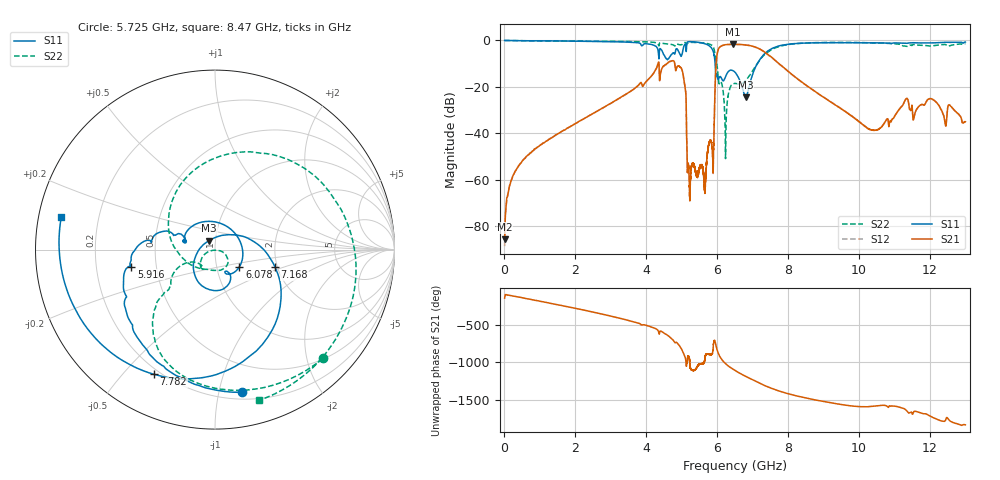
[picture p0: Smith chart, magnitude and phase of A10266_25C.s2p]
!Akoustis s2p Touchstone File
!Script Version: 1.0
!Creation Data: 12/28/2021 at 11:15 AM
!DEEMBEDDING STATE: ON
!DEMBEDDING OFFSET: 0.4 dB static
! Freq Mag(S11) Angle(S11)Mag(S21) Angle(S21)Mag(S12) Angle(S12)Mag(S22) Angle(S22)
# GHz S MA R 50
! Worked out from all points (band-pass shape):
!   11000 points, 10 MHz to 13 GHz, reference 50 ohm
!   highest |S21| = -1.69 dB at 6.448 GHz (marker M1); lowest = -85.7 dB at 10 MHz (marker M2)
!   |S21| within 3 dB of the highest: 6.019 GHz to 7.311 GHz (1.292 GHz wide, 19.4 % of centre)
!   lowest |S11| = -24.5 dB at 6.805 GHz (marker M3), VSWR 1.13, Z = 46.7 + j4.66 ohm
!   |S11| at or under -10 dB: 5.944 GHz to 7.137 GHz (1.192 GHz wide, 18.2 % of centre)
!   |S22| runs from -51.0 to 0.0 dB; largest |S21 - S12| = 0.0056
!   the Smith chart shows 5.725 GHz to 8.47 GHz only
!   S11 on the Smith chart (normalised r, x): 5.725 GHz: 0.26, -1.18; 5.916 GHz: 0.36, -0.09; 6.078 GHz: 1.29, -0.25; 7.168 GHz: 1.94, -0.42; 7.782 GHz: 0.18, -0.61; 8.47 GHz: 0.07, +0.11
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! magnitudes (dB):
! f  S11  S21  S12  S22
! 10 MHz  0.0  -85.7  -88.7  0.0
! 50.1 MHz  0.0  -71.4  -71.9  0.0
! 110.3 MHz  -0.1  -65.7  -65.9  -0.1
! 370.9 MHz  -0.1  -54.9  -54.8  -0.1
! 1.193 GHz  -0.2  -43.4  -43.3  -0.2
! 3.94 GHz  -1.5  -19.0  -19.0  -0.6
! 4.972 GHz  -6.5  -11.7  -11.7  -1.9
! 5.107 GHz  -1.6  -21.2  -21.2  -1.0
! 5.229 GHz  -0.5  -68.0  -67.1  -0.9
! 5.654 GHz  -1.4  -63.8  -63.8  -1.2
! 5.725 GHz  -1.8  -49.0  -48.9  -1.4
! 5.916 GHz  -6.5  -36.4  -36.4  -3.8
! 5.976 GHz  -15.2  -9.4  -9.4  -9.4
! 6.078 GHz  -15.6  -2.8  -2.9  -18.2
! 6.239 GHz  -15.6  -1.8  -1.8  -50.0
! 6.448 GHz  -13.0  -1.7  -1.7  -18.8
! 6.805 GHz  -24.5  -2.0  -1.9  -17.3
! 7.168 GHz  -9.2  -3.5  -3.5  -9.2
! 7.782 GHz  -2.2  -10.5  -10.6  -2.5
! 8.47 GHz  -1.1  -18.9  -18.9  -1.2
! 10.31 GHz  -1.0  -38.4  -38.3  -1.0
! 13 GHz  -0.7  -35.0  -34.9  -1.5
